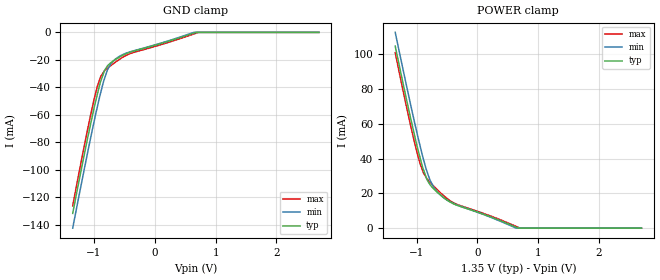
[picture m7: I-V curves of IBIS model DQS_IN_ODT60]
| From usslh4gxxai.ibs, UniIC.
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| MODEL DQS_IN_ODT60 (Data Strobe Input with 60ohm ODT, 800-2133Mbps)
[Model]   DQS_IN_ODT60
Model_type   Input
Vinl = 545.000mV
Vinh = 805.000mV
|   typ   min   max
|C_comp   1.069pF   1.013pF   1.108pF
C_comp_power_clamp   0.5345pF   0.5065pF   0.5540pF
C_comp_gnd_clamp   0.5345pF   0.5065pF   0.5540pF
| Note: C_comp changes when the ODT circuit is enabled.
[Model Spec]
| Input threshold voltage corners
Vinl   0.5450V   0.5115V   0.5825V
Vinh   0.8050V   0.7715V   0.8425V
| Dynamic Overshoot Parameters from DDR3L Specification
|D_overshoot_ampl_h   0.40   NA   NA
|D_overshoot_ampl_l   0.40   NA   NA
|D_overshoot_area_h   0.11n   NA   NA
|D_overshoot_area_l   0.11n   NA   NA
[Receiver Thresholds]
|Vth   =  0.675V
|Vth_min  =  0.6615V
|Vth_max  =  0.6885V
|Vinh_ac  =  0.130V
|Vinh_dc  =  0.090V
|Vinl_ac  = -0.130V
|Vinl_dc  = -0.090V
|Tslew_ac =  5.000ns |Not specified, so set to high value
|Threshold_sensitivity = 0.50
|Reference_supply Power_clamp_ref
|NOTE: If using the IBISCHK 4.2.1 or older parser, Differential receiver
|threshold parameters must be commented out because the parser generates
|errors for multiple differential models.
Vcross_low   = 0.545V
Vcross_high  = 0.805V
Vdiff_ac   = 260mV
Vdiff_dc   = 180mV
Tdiffslew_ac = 10.000ns |Not specified, so set to high value
[Voltage Range]   1.3500V   1.2830V   1.4250V
[POWER Clamp Reference]   1.3500V   1.2830V   1.4250V
[Temperature Range]   45.0   95.0   -40.0
[GND Clamp]
|   Voltage   I(typ)   I(min)   I(max)
-1.35V    -131.8mA   -142.6mA   -126.3mA
-1.11V    -77.97mA   -88.53mA   -71.57mA
-1V       -55.11mA   -65.16mA   -48.92mA
-945mV    -45.04mA   -54.11mA   -39.28mA
-885mV    -35.01mA   -42.95mA   -31.73mA
-825mV    -27.52mA   -33.34mA   -27.93mA
-780mV    -24.5mA    -27.42mA   -26.15mA
-715mV    -21.84mA   -22.34mA   -23.89mA
-650mV    -19.84mA   -19.53mA   -21.78mA
-410mV    -14.49mA   -14.22mA   -15.53mA
720mV     0A         0A         0A
2.7V      0A         0A         0A
[POWER Clamp]
|   Voltage   I(typ)   I(min)   I(max)
-1.35V    104.7mA    112.7mA    101mA
-1.11V    65.25mA    73.14mA    61.03mA
-1V       48.43mA    55.95mA    44.61mA
-940mV    40.31mA    47.08mA    36.96mA
-885mV    33.51mA    39.51mA    31.67mA
-830mV    28.17mA    32.8mA     28.48mA
-780mV    25.15mA    27.73mA    26.46mA
-715mV    22.52mA    23.42mA    24.08mA
-560mV    17.79mA    17.7mA     18.9mA
-335mV    13.18mA    13.33mA    13.68mA
705mV     0A         0A         0A
2.7V      0A         0A         0A
